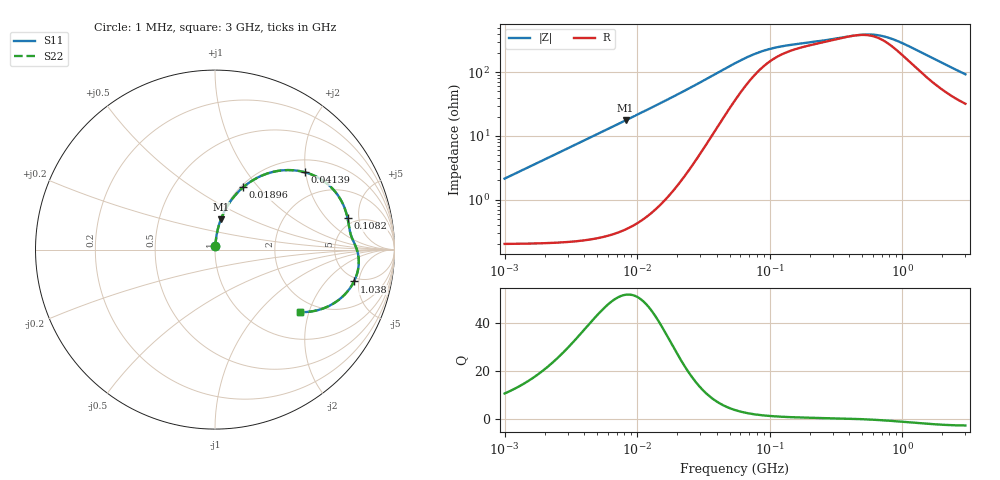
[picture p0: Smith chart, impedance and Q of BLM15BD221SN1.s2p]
! BLM15BD221SN1
# Hz S RI R 50
!Freq.(Hz) S11(Real) S11(Imag) S21(Real) S21(Imag) S12(Real) S12(Imag) S22(Real) S22(Imag)
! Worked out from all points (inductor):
!   401 points, 1 MHz to 3 GHz, reference 50 ohm
!   read as one part in series: L = 339 nH near 1.041 MHz
!   highest Q = 51.5 at 8.18 MHz (marker M1), where L = 341 nH
!   self-resonance near 439.1 MHz
!   S11 on the Smith chart (normalised r, x): 1 MHz: 1.00, +0.04; 18.96 MHz: 1.03, +0.84; 41.39 MHz: 1.30, +1.99; 108.2 MHz: 4.28, +3.54; 1.038 GHz: 4.47, -4.31; 3 GHz: 1.64, -1.74
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1000000  0.00246 0.0212  0.9975 -0.0212  0.9975 -0.0212  0.00246 0.0212
2097170  0.00405 0.0444  0.9959 -0.0444  0.9959 -0.0444  0.00405 0.0444
3823119  0.00882 0.0806  0.9912 -0.0806  0.9912 -0.0806  0.00882 0.0806
8179831  0.0329 0.169  0.9671 -0.169  0.9671 -0.169  0.0329 0.169
1.461624e7  0.0978 0.285  0.9022 -0.285  0.9022 -0.285  0.0978 0.285
1.896016e7  0.1578 0.3479  0.8422 -0.3479  0.8422 -0.3479  0.1578 0.3479
2.362996e7  0.2315 0.3982  0.7685 -0.3982  0.7685 -0.3982  0.2315 0.3982
2.944989e7  0.328 0.434  0.672 -0.434  0.672 -0.434  0.328 0.434
3.526298e7  0.4194 0.4429  0.5806 -0.4429  0.5806 -0.4429  0.4194 0.4429
4.138676e7  0.5023 0.4304  0.4977 -0.4304  0.4977 -0.4304  0.5023 0.4304
5.477226e7  0.6253 0.3668  0.3747 -0.3668  0.3747 -0.3668  0.6253 0.3668
7.395247e7  0.7028 0.2734  0.2972 -0.2734  0.2972 -0.2734  0.7028 0.2734
1.081723e8  0.7386 0.1751  0.2614 -0.1751  0.2614 -0.1751  0.7386 0.1751
2.094008e8  0.7571 0.0814  0.2429 -0.0814  0.2429 -0.0814  0.7571 0.0814
5.154121e8  0.797 -0.025  0.203 0.025  0.203 0.025  0.797 -0.025
6.423554e8  0.8012 -0.0659  0.1988 0.0659  0.1988 0.0659  0.8012 -0.0659
8.005644e8  0.7965 -0.1141  0.2035 0.1141  0.2035 0.1141  0.7965 -0.1141
1.038491e9  0.7745 -0.1776  0.2255 0.1776  0.2255 0.1776  0.7745 -0.1776
1.402151e9  0.7217 -0.2515  0.2783 0.2515  0.2783 0.2515  0.7217 -0.2515
1.893158e9  0.6381 -0.3125  0.3619 0.3125  0.3619 0.3125  0.6381 -0.3125
2.407135e9  0.5543 -0.3416  0.4457 0.3416  0.4457 0.3416  0.5543 -0.3416
3e9  0.4724 -0.3482  0.5276 0.3482  0.5276 0.3482  0.4724 -0.3482
